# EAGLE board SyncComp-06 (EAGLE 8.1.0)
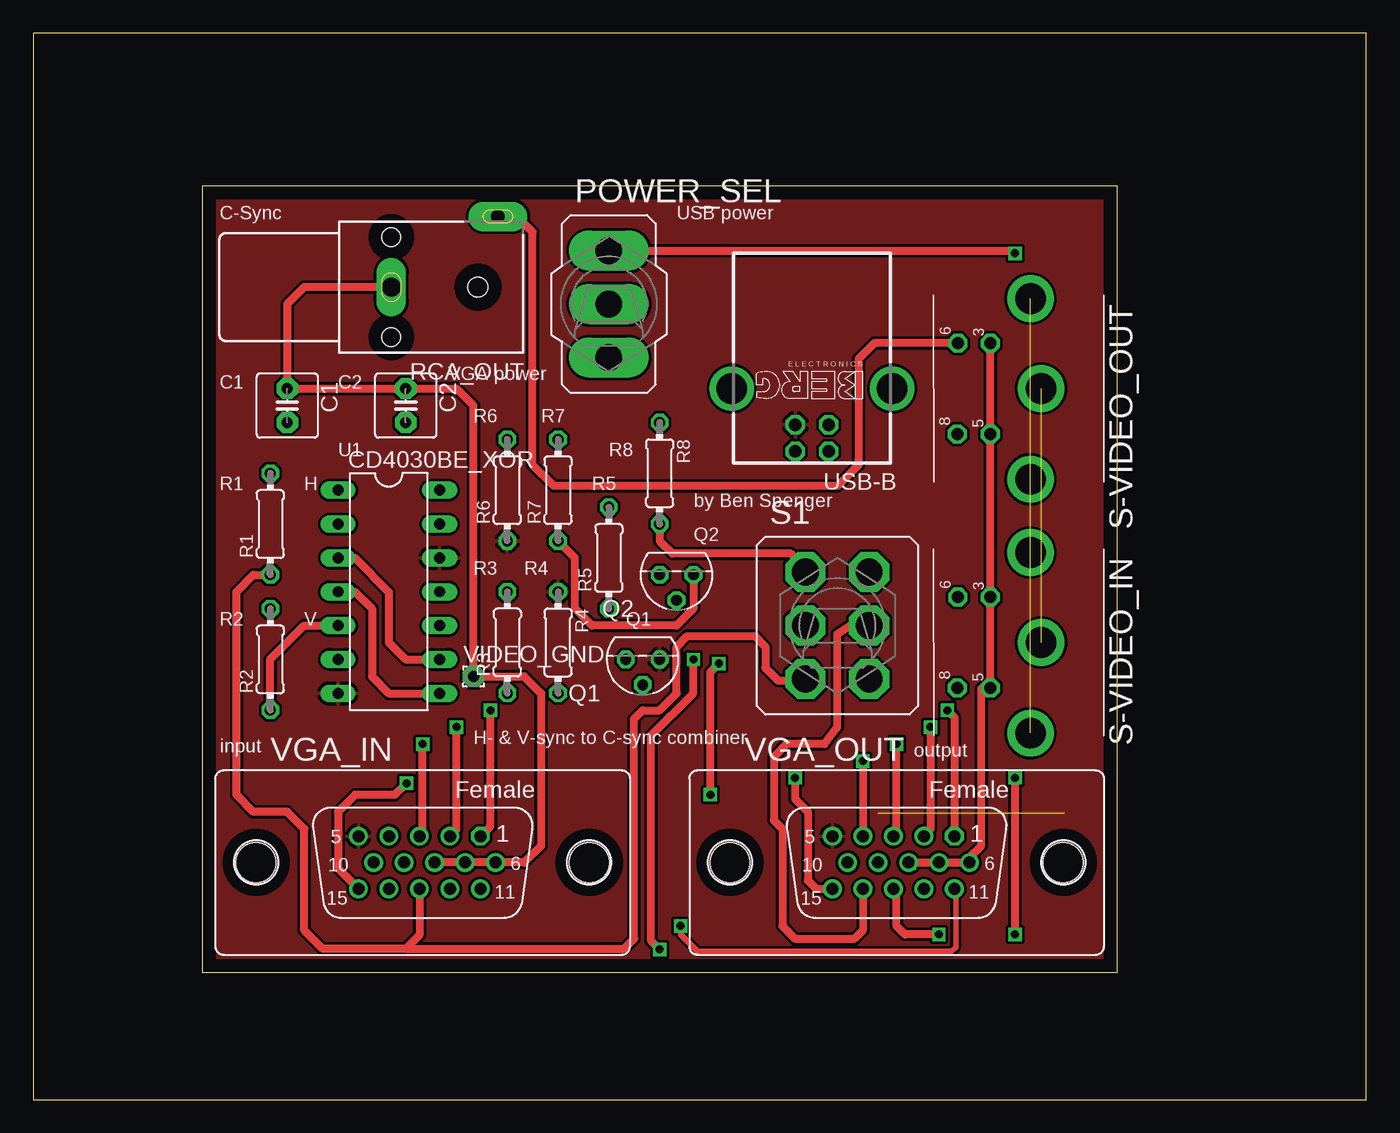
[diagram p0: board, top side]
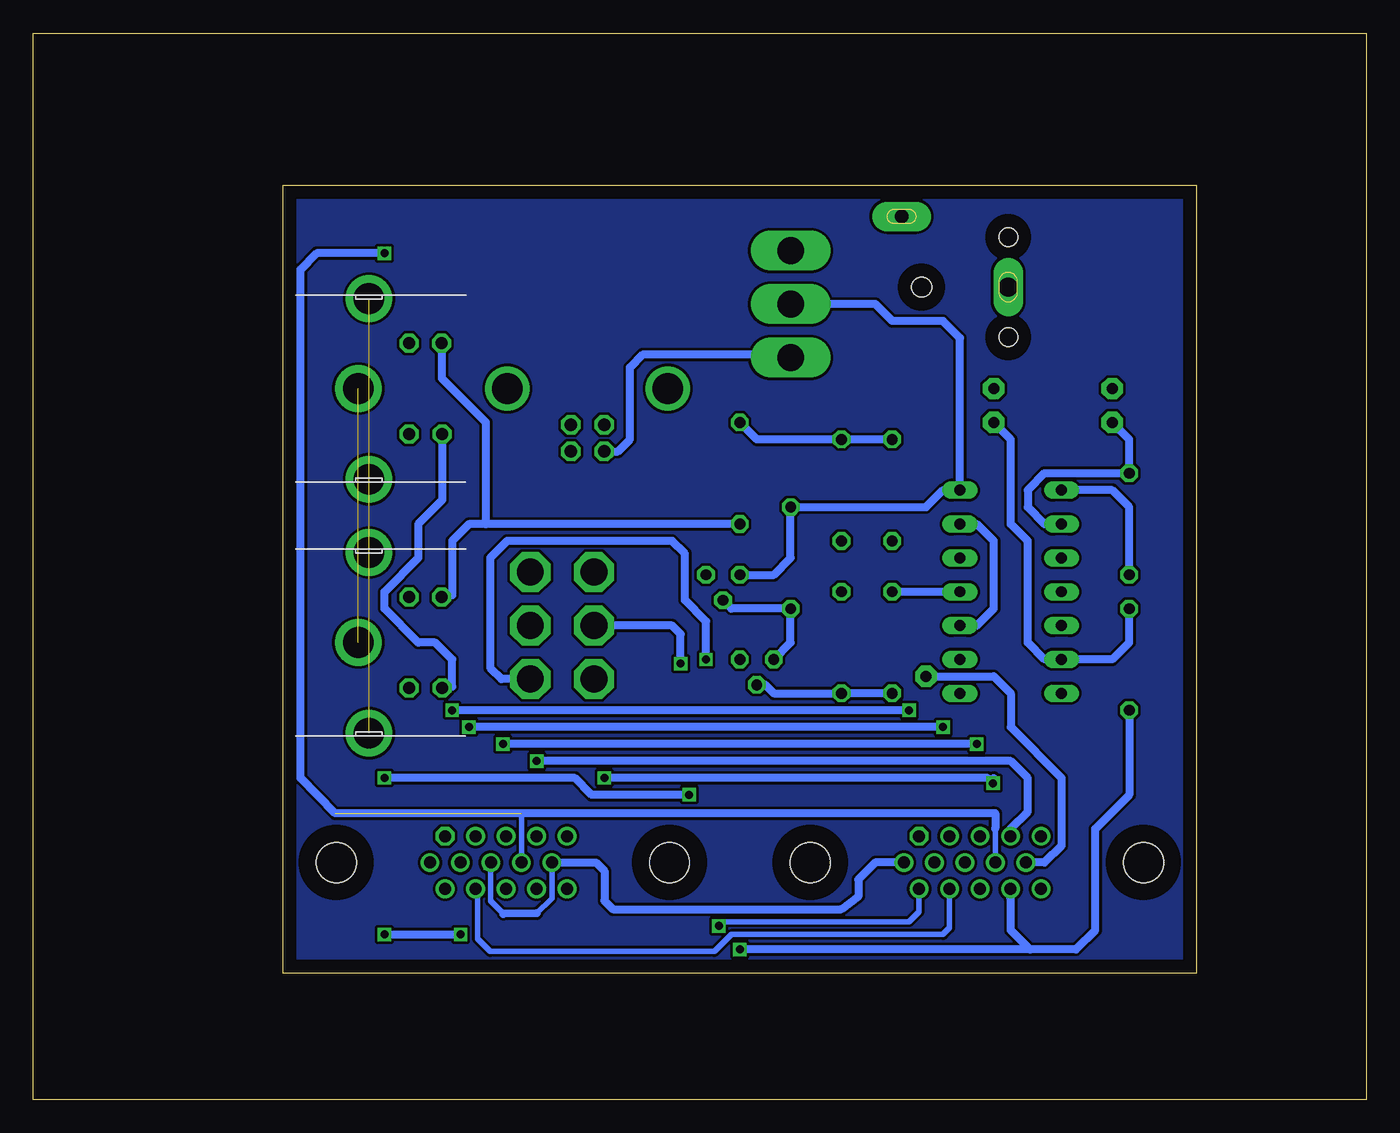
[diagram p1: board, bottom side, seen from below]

Size 100 x 80 mm. Coordinates in mm from the lower left corner, seen from the top.
Outline: 0,0 100,0 100,80 0,80 0,0
Outline: 12.7,68.58 81.28,68.58 81.28,9.53 12.7,9.53 12.7,68.58
Copper layers (1*16): Top 0.035mm / dielectric 1.5mm / Bottom 0.035mm
Design rules "default": minimum track width 10mil, minimum drill 24mil, track to track 8mil, track to pad 8mil, pad to pad 8mil, via to via 8mil, smd to smd 8mil, copper to edge 40mil, drill to drill 8mil, minimum pad ring 10mil, minimum via ring 8mil, stop-mask expansion 4mil, vias tented up to drill 0mil, thermal gap 10mil

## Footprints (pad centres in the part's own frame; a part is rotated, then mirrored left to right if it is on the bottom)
C2.5-5 = drill 0.813 pad 1.6 octagon: 1 -1.27,0; 2 1.27,0
DIL14 = drill 0.813 long: 1 -7.62,-3.81; 2 -5.08,-3.81; 3 -2.54,-3.81; 4 0,-3.81; 5 2.54,-3.81; 6 5.08,-3.81; 7 7.62,-3.81; 8 7.62,3.81; 9 5.08,3.81; 10 2.54,3.81; 11 0,3.81; 12 -2.54,3.81; 13 -5.08,3.81; 14 -7.62,3.81
320-916 = drill 2.007 long: 1 0,4.013; 2 0,0; 3 0,-4.013
TO92D = drill 0.813 octagon: B 0,1.905; C 1.27,0; E -1.27,0
0204/7 = drill 0.813 octagon: 1 -3.81,0; 2 3.81,0
WBTOR1 = drill 1.4 pad 2.2 long: S 0,-4 | drill 1 pad 2.2 long: T 5.3,-12 | hole 1.4: -3.75,-4; 3.75,-4 | hole 1.5: 0,-10.5
320-938 = drill 2.007 octagon: 1 -2.388,4.013; 2 -2.388,0; 3 -2.388,-4.013; 4 2.388,4.013; 5 2.388,0; 6 2.388,-4.013
M_DIN4 = drill 0.9 pad 1.422 octagon: 3 -3.4,-3.75; 5 3.4,-3.75; 6 -3.4,-6.2; 8 3.4,-6.25 | drill 2.3 pad 3.5: SH1 6.8,-0.75; SH2 0,0.05; SH3 -6.75,-0.75
PN61729-S = drill 0.95 octagon: 1 1.25,4.71; 2 -1.25,4.71; 3 -1.25,2.71; 4 1.25,2.71 | drill 2.3 pad 2.9: S1 -6.02,0; S2 6.02,0
HDF15V = drill 0.9 octagon: 1 4.329,1.98 | drill 0.9: 2 2.043,1.98; 3 -0.243,1.98; 4 -2.529,1.98; 5 -4.815,1.98; 6 5.472,0; 7 3.186,0; 8 0.9,0; 9 -1.386,0; 10 -3.672,0; 11 4.329,-1.98; 12 2.043,-1.98; 13 -0.243,-1.98; 14 -2.529,-1.98; 15 -4.815,-1.98 | hole 3: -12.5,0; 12.5,0
1,6/0,8 = drill 0.813 pad 1.6 octagon: 1 0,0

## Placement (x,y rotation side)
C1  22 uF  [C2.5-5]  19.05,52.07 270 top
C2  22 uF  [C2.5-5]  27.94,52.07 270 top
CD4030BE_XOR  [DIL14]  26.67,38.1 270 top
POWER_SEL  [320-916]  43.18,59.69 0 top
Q1  2N3904  [TO92D]  45.72,33.02 180 top
Q2  2N3904  [TO92D]  48.26,39.37 180 top
R1  2.2 kOhm  [0204/7]  17.78,43.18 90 top
R2  2.2 kOhm  [0204/7]  17.78,33.02 90 top
R3  2.2 kOhm  [0204/7]  35.56,34.29 90 top
R4  2.2 kOhm  [0204/7]  39.37,34.29 270 top
R5  2.2 kOhm  [0204/7]  43.18,40.64 90 top
R6  47 Ohm  [0204/7]  35.56,45.72 90 top
R7  47 Ohm  [0204/7]  39.37,45.72 90 top
R8  47 Ohm  [0204/7]  46.99,46.99 270 top
RCA_OUT  WBTOR1  [WBTOR1]  22.86,60.96 90 top
S1  [320-938]  60.33,35.56 0 top
S-VIDEO_IN  [M_DIN4]  75.56,34.29 270 top
S-VIDEO_OUT  [M_DIN4]  75.56,53.34 270 top
USB-B  PN61729-S  [PN61729-S]  58.42,53.34 180 top
VGA_IN  [HDF15V]  29.21,17.78 0 top
VGA_OUT  [HDF15V]  64.77,17.78 0 top
VIDEO_GND  [1,6/0,8]  33.02,31.75 0 top

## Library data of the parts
C1 C2 = capacitor-wima
CD4030BE_XOR = ic-package
POWER_SEL S1 = switch
Q1 Q2 = transistor-small-signal
R1-R8 = resistor
RCA_OUT = con-lumberg; MPN: WBTOR 1 BLACK; OC_FARNELL: 1200146; OC_NEWARK: 98K2588
S-VIDEO_IN S-VIDEO_OUT = mini_din
USB-B = con-berg; OC_FARNELL: unknown; OC_NEWARK: unknown
VGA_IN VGA_OUT = con-subd; OC_FARNELL: unknown; OC_NEWARK: unknown
VIDEO_GND = wirepad

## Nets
GND: CD4030BE_XOR.7 CD4030BE_XOR.12 Q1.E R4.1 R6.1 USB-B.4 VGA_IN.5 VGA_OUT.5
N$1: POWER_SEL.3 USB-B.1
N$2: POWER_SEL.1 VGA_IN.9 VGA_OUT.9
N$3: C1.2 CD4030BE_XOR.2 R1.2
N$4: VGA_IN.15 VGA_OUT.15
N$5: CD4030BE_XOR.5 R2.1 S1.6 VGA_IN.14
N$6: C2.2 CD4030BE_XOR.6 R2.2
N$7: CD4030BE_XOR.4 CD4030BE_XOR.8
N$8: CD4030BE_XOR.3 CD4030BE_XOR.9
N$9: CD4030BE_XOR.10 CD4030BE_XOR.13
N$10: VGA_IN.11 VGA_OUT.11
N$11: CD4030BE_XOR.14 POWER_SEL.2 Q2.C R5.2
N$12: VGA_IN.12 VGA_OUT.12
N$13: CD4030BE_XOR.11 R3.2
N$14: Q1.B R3.1 R4.2
N$15: Q1.C Q2.B R5.1
N$16: CD4030BE_XOR.1 R1.1 S1.3 VGA_IN.13
N$17: VGA_IN.1 VGA_OUT.1
N$18: VGA_IN.2 VGA_OUT.2
N$19: R8.2 RCA_OUT.T S1.1 S-VIDEO_IN.6 S-VIDEO_OUT.6
N$20: R6.2 R7.2 R8.1
N$21: Q2.E R7.1
N$22: VGA_IN.3 VGA_OUT.3
N$23: VGA_IN.4 VGA_OUT.4
N$24: C1.1 C2.1 RCA_OUT.S S-VIDEO_IN.3 S-VIDEO_IN.5 S-VIDEO_OUT.3 S-VIDEO_OUT.5 VGA_IN.6 VGA_IN.7 VGA_IN.8 VGA_IN.10 VGA_OUT.6 VGA_OUT.7 VGA_OUT.8 VGA_OUT.10 VIDEO_GND.1
N$26: S1.5 VGA_OUT.14
N$28: S-VIDEO_IN.8 S-VIDEO_OUT.8
N$30: S1.2 VGA_OUT.13
PE1: S-VIDEO_IN.SH1 S-VIDEO_OUT.SH1
PE2: S-VIDEO_IN.SH2 S-VIDEO_OUT.SH2
PE3: S-VIDEO_IN.SH3 S-VIDEO_OUT.SH3

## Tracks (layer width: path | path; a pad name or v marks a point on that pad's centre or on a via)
GND
  pour Top (isolate 0.15): 12.7,68.58 81.28,68.58 81.28,9.53 12.7,9.53
N$1
  Bottom 0.61: POWER_SEL.3 43.38,55.88 54.29,55.88 55.24,54.93 55.24,49.53 56.15,48.63 USB-B.1
N$2  (via drill 0.6)  (1 unrouted)
  Top 0.61: POWER_SEL.1 73.46,63.7 v73.66,63.5
  Bottom 0.406: 63.38,21.47 VGA_OUT.9 | 27.82,20.33 VGA_IN.9 | 27.94,21.59 27.82,21.47
  Bottom 0.61: 27.82,20.33 27.82,21.47 77.35,21.47 79.96,24.13 79.96,62.28 78.74,63.5 v73.66,63.5
N$3
  Bottom 0.61: CD4030BE_XOR.2 24.13,43.18 25.4,44.45 25.4,45.72 24.13,46.99 R1.2 17.78,49.53 C1.2
N$4  (via drill 0.6)
  Top 0.61: VGA_IN.15 22.86,17.34 22.86,21.59 24.13,22.86 27.12,22.86 v27.99,23.73 | VGA_OUT.15 58.74,15.8 58.1,16.43 58.1,21.59 57.15,22.54 v57.15,24.13
  Bottom 0.61: 27.94,24.13 27.94,23.78 v27.99,23.73 28.39,24.13 v57.15,24.13
N$5  (via drill 0.6)
  Top 0.61: v46.99,11.25 46.35,11.89 46.35,27.3 49.53,30.48 v49.53,33.02 | R2.1 17.78,33.02 20.32,35.56 CD4030BE_XOR.5
  Bottom 0.61: 25.22,11.25 v46.99,11.25 | VGA_IN.14 26.68,15.07 26.67,15.06 26.67,12.7 25.22,11.25 | 25.22,11.25 21.77,11.25 20.32,12.7 20.32,20.32 17.78,22.86 R2.1 | v49.53,33.02 49.53,35.88 51.12,37.47 51.12,40.96 52.07,41.91 64.45,41.91 65.72,40.64 65.72,32.38 64.88,31.55 S1.6
N$6
  Bottom 0.61: R2.2 17.78,34.29 19.05,33.02 CD4030BE_XOR.6 24.13,33.02 25.4,34.29 25.4,41.91 26.67,43.18 26.67,49.53 C2.2
N$7
  Top 0.61: CD4030BE_XOR.4 24.13,38.1 25.4,36.83 25.4,31.75 26.67,30.48 CD4030BE_XOR.8
N$8
  Top 0.61: CD4030BE_XOR.3 24.13,40.64 26.67,38.1 26.67,34.29 27.94,33.02 CD4030BE_XOR.9
N$9
  Bottom 0.61: CD4030BE_XOR.10 29.21,35.56 27.94,36.83 27.94,41.91 29.21,43.18 CD4030BE_XOR.13
N$10  (via drill 0.6)
  Top 0.406: v48.57,13.01 48.57,12.39 49.85,11.11 68.9,11.11 69.22,11.43 69.22,15.68 VGA_OUT.11
  Bottom 0.406: VGA_IN.11 33.54,14.09 34.29,13.34 48.25,13.34 v48.57,13.01
N$11
  Bottom 0.61: Q2.C 44.45,39.37 43.18,40.64 R5.2 33.02,44.45 31.75,45.72 CD4030BE_XOR.14 30.48,57.15 31.75,58.42 35.56,58.42 36.83,59.69 POWER_SEL.2
N$12
  Bottom 0.406: VGA_IN.12 31.25,12.88 31.75,12.38 47.62,12.38 48.9,11.11 65.72,11.11 66.67,12.06 66.67,15.66 VGA_OUT.12
N$13
  Bottom 0.61: CD4030BE_XOR.11 R3.2
N$14
  Bottom 0.61: R3.1 R4.2 44.45,30.48 45.09,31.11 Q1.B
N$15
  Bottom 0.61: Q1.C 43.18,34.29 R5.1 47.62,36.83 Q2.B
N$16
  Top 0.61: R1.1 16.51,39.37 15.24,38.1 15.24,22.86 16.51,21.59 19.05,21.59 20.32,20.32 20.32,12.7 21.71,11.31 27.94,11.31 | VGA_IN.13 28.97,12.34 27.94,11.31 | 27.94,11.31 44.33,11.31 45.09,12.06 45.09,28.57 45.72,29.21 46.99,29.21 48.26,30.48 48.26,33.97 49.05,34.77 52.07,34.77 | 57.94,31.6 S1.3 57.82,31.43 55.88,31.43 54.93,32.38 54.93,33.97 54.13,34.77 52.07,34.77 | 52.07,34.77 52.23,34.77
  Bottom 0.61: CD4030BE_XOR.1 19.05,45.72 17.78,44.45 R1.1
N$17  (via drill 0.6)
  Top 0.61: VGA_IN.1 34.29,20.51 v34.29,29.21 | v68.58,29.21 69.1,28.69 VGA_OUT.1
  Bottom 0.61: v34.29,29.21 v68.58,29.21
N$18  (via drill 0.6)
  Top 0.61: VGA_IN.2 31.75,20.26 v31.75,27.94 | v67.31,27.94 67.31,20.32 66.81,19.82 VGA_OUT.2
  Bottom 0.61: v31.75,27.94 v67.31,27.94
N$19
  Top 0.61: R8.2 46.99,41.91 47.94,40.96 56.83,40.96 S1.1 | S-VIDEO_OUT.6 63.09,56.74 61.91,55.56 61.91,47.62 60.33,46.04 39.05,46.04 37.47,47.62 37.47,65.09 36.2,66.36 34.96,66.36 RCA_OUT.T
  Bottom 0.61: R8.2 66.04,43.18 | 66.04,43.18 67.31,43.18 68.58,41.91 68.58,37.84 S-VIDEO_IN.6 | 66.04,43.18 66.04,50.8 69.36,54.12 S-VIDEO_OUT.6
N$20
  Bottom 0.61: R6.2 R7.2 45.72,49.53 R8.1
N$21
  Top 0.61: Q2.E 49.53,36.83 48.26,35.56 41.91,35.56 40.64,36.83 40.64,40.64 R7.1
N$22  (via drill 0.6)
  Top 0.61: VGA_IN.3 29.21,20 v29.21,26.67 | VGA_OUT.3 64.77,20 v64.77,26.67
  Bottom 0.61: v29.21,26.67 v64.77,26.67
N$23  (via drill 0.6)
  Top 0.61: v62.23,25.4 62.24,25.39 VGA_OUT.4
  Bottom 0.61: v62.23,25.4 26.67,25.4 25.4,24.13 25.4,21.59 26.68,20.31 VGA_IN.4
N$24  (via drill 0.6)
  Top 0.406: v65.7,17.75 VGA_OUT.8
  Top 0.61: VGA_IN.6 VGA_IN.7 VGA_IN.8 | VGA_IN.6 34.68,18.17 | VGA_OUT.8 VGA_OUT.7 VGA_OUT.6 70.24,18.17 71.12,19.05 71.12,30.83 S-VIDEO_IN.5 S-VIDEO_IN.3 S-VIDEO_OUT.5 S-VIDEO_OUT.3 | RCA_OUT.S 20.32,60.96 19.05,59.69 C1.1 C2.1 31.75,53.34 33.02,52.07 VIDEO_GND.1 36.83,31.75 38.1,30.48 38.1,19.05 36.83,17.78 VGA_IN.6
  Bottom 0.406: VGA_OUT.10 61.1,15.1 62.23,13.97 | 64.72,13.92 65.7,14.9 v65.7,17.75
  Bottom 0.61: VIDEO_GND.1 27.94,31.75 26.67,30.48 26.67,27.94 22.86,24.13 22.86,19.05 24.13,17.78 VGA_IN.10 | VGA_IN.6 36.83,17.78 38.1,16.51 38.1,15.24 39.37,14.29 56.52,14.29 57.15,14.92 57.15,17.14 57.78,17.78 VGA_OUT.10 | 62.23,13.97 64.72,13.92
N$25
  pour Bottom (isolate 0.15): 12.7,68.58 81.28,68.58 81.28,9.53 12.7,9.53
N$26
  Top 0.61: VGA_OUT.14 62.24,12.71 61.59,12.06 57.15,12.06 56.2,13.02 56.2,20.32 55.56,20.95 55.56,25.72 56.52,26.67 59.37,26.67 60.33,27.94 60.33,34.92 61.28,35.56 S1.5
N$28
  Bottom 0.61: S-VIDEO_IN.8 68.58,30.99 68.58,33.02 69.85,34.29 71.12,34.29 73.66,36.83 73.66,38.1 71.12,40.64 71.12,43.18 69.31,44.98 S-VIDEO_OUT.8
N$30  (via drill 0.6)
  Top 0.61: v50.8,22.86 50.8,32.07 v51.44,32.7 | v73.66,24.13 v73.66,12.38 | v67.94,12.38 65.41,12.38 64.77,13.02 64.77,15.56 VGA_OUT.13
  Bottom 0.61: v50.8,22.86 58.1,22.86 59.37,24.13 v73.66,24.13 | v73.66,12.38 v67.94,12.38 | v51.44,32.7 51.44,34.92 52.07,35.56 S1.2
PE1  (1 unrouted)
PE2  (1 unrouted)
PE3  (1 unrouted)

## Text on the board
tPlace: C-Sync | USB power | VGA power | C1 | C2 | R6 | R7 | U1 | R8 | R1 | H | R5 | by Ben Spenger | Q2 | R3 | R4 | R2 | V | Q1 | H- & V-sync to C-sync combiner | input | output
